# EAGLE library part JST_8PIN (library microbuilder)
JST 8-Pin Right-Angle Connector
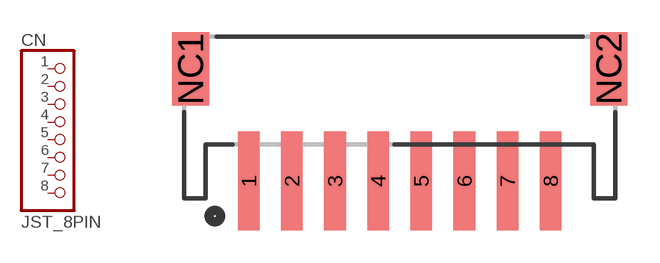
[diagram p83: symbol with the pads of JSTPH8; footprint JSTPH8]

Designator prefix CN

## JST_8PIN  [JSTPH8]
1  1  pas
2  2  pas
3  3  pas
4  4  pas
5  5  pas
6  6  pas
7  7  pas
8  8  pas

## Footprint JSTPH8 (pad centres in mm)
smd 1 x 4.6: 1 -7,-3.7; 2 -5,-3.7; 3 -3,-3.7; 4 -1,-3.7; 5 1,-3.7; 6 3,-3.7; 7 5,-3.7; 8 7,-3.7
smd 1.7 x 3.4: NC1 -9.7,1.5; NC2 9.7,1.5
